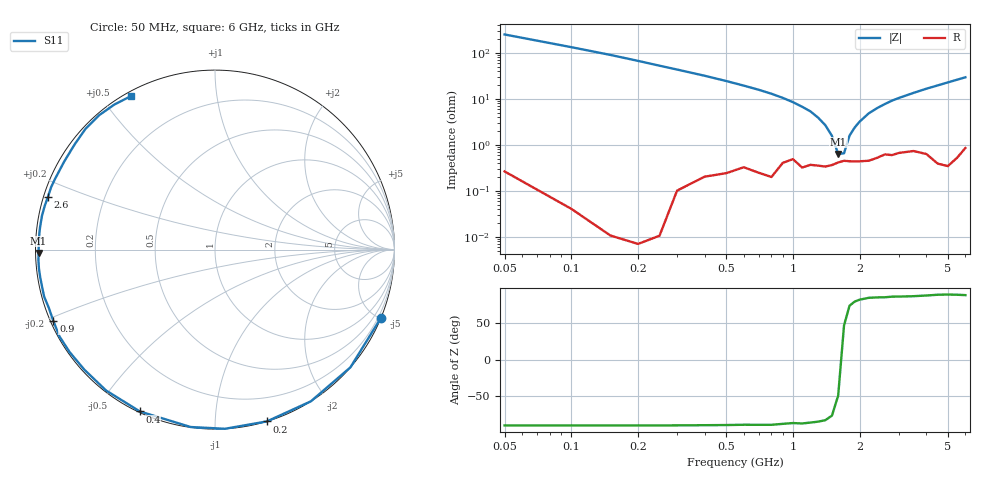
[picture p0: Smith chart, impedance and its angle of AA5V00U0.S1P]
! Infineon Technologies  Discrete & RF Semiconductors
! BBY66-02W
! Si Tuning Diode in SCD-80
! VR = 5 V
! S-Parameters:  June  2000
# GHz  S  MA  R  50
!  f  S11
! GHz  MAG  ANG
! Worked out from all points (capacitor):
!   34 points, 50 MHz to 6 GHz, reference 50 ohm
!   read as one part to ground: C = 11.9 pF near 50 MHz
!   lowest |Z| = 635 mohm at 1.6 GHz (marker M1)
!   series resonance near 1.65 GHz, so ESL is about 780 pH
!   S11 on the Smith chart (normalised r, x): 50 MHz: 0.01, -5.05; 200 MHz: 0.00, -1.35; 400 MHz: 0.00, -0.64; 900 MHz: 0.01, -0.21; 2.6 GHz: 0.01, +0.15; 6 GHz: 0.02, +0.59
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0.05  0.9996 -22.4
0.1  0.9998 -41.0
0.15  0.9999 -57.7
0.2  0.9999 -73.2
0.25  0.9998 -86.8
0.3  0.9977 -97.8
0.4  0.9942 -114.9
0.5  0.9922 -127.7
0.6  0.9887 -137.4
0.7  0.991 -144.8
0.8  0.9925 -150.9
0.9  0.9845 -156.2
1  0.9811 -160.7
1.1  0.9874 -164.6
1.3  0.986 -171.1
1.4  0.9866 -173.9
1.6  0.9835 -178.9
1.8  0.9825 176.5
2.2  0.9822 168.9
2.4  0.9795 165.6
2.6  0.976 162.4
2.8  0.977 159.2
3.5  0.9729 149.7
4  0.9774 143.1
4.5  0.9865 137.0
5  0.9886 130.8
5.5  0.9837 124.7
6  0.9749 118.8
